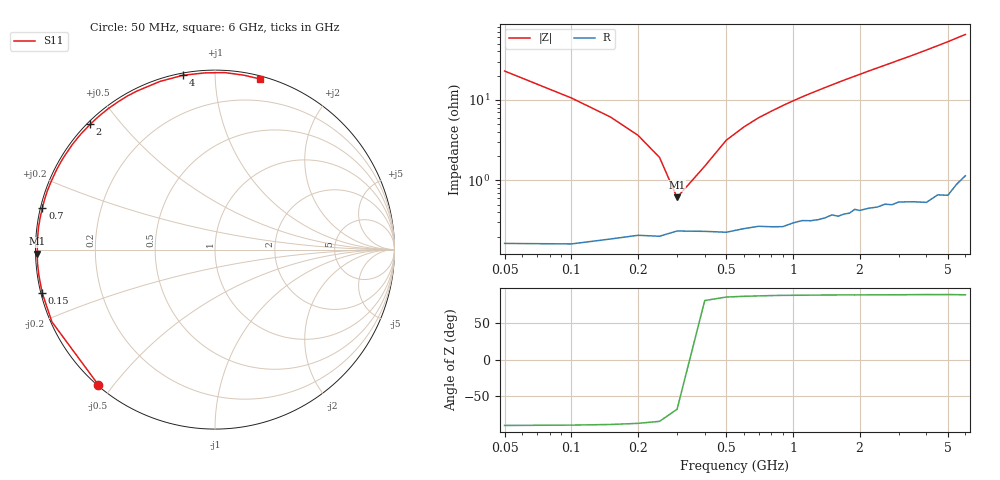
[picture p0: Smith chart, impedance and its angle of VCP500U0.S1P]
! Infineon Technologies  Discrete & RF Semiconductors
! BBY 56-03
! Si Tuning Diode in SOD323
! VR = 0.5 V
! S-Parameters:  June  1999
# GHz  S  MA  R  50
!  f  S11
! GHz  MAG  ANG
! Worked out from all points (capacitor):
!   34 points, 50 MHz to 6 GHz, reference 50 ohm
!   read as one part to ground: C = 136 pF near 50 MHz
!   lowest |Z| = 614 mohm at 300 MHz (marker M1)
!   series resonance near 327.7 MHz, so ESL is about 1.7 nH
!   S11 on the Smith chart (normalised r, x): 50 MHz: 0.00, -0.46; 150 MHz: 0.00, -0.12; 700 MHz: 0.01, +0.12; 2 GHz: 0.01, +0.42; 4 GHz: 0.01, +0.83; 6 GHz: 0.02, +1.30
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0.05  0.9946 -130.9
0.1  0.9938 -156.1
0.15  0.9927 -166.0
0.2  0.9918 -171.7
0.25  0.9919 -175.6
0.3  0.9906 -178.7
0.4  0.9907 176.6
0.5  0.991 172.8
0.7  0.9895 166.3
0.8  0.9897 163.5
0.9  0.9897 160.7
1  0.9887 158.0
1.2  0.9881 152.9
1.4  0.9874 148.1
1.6  0.9871 143.5
1.7  0.9865 141.2
2  0.9857 134.9
2.2  0.9852 130.8
2.4  0.9852 127.0
2.6  0.9844 123.3
2.8  0.9852 119.7
3  0.9846 116.2
3.5  0.9859 108.1
4  0.9875 100.4
4.5  0.9861 93.3
5  0.9877 86.8
5.5  0.9849 80.6
6  0.9832 75.1
